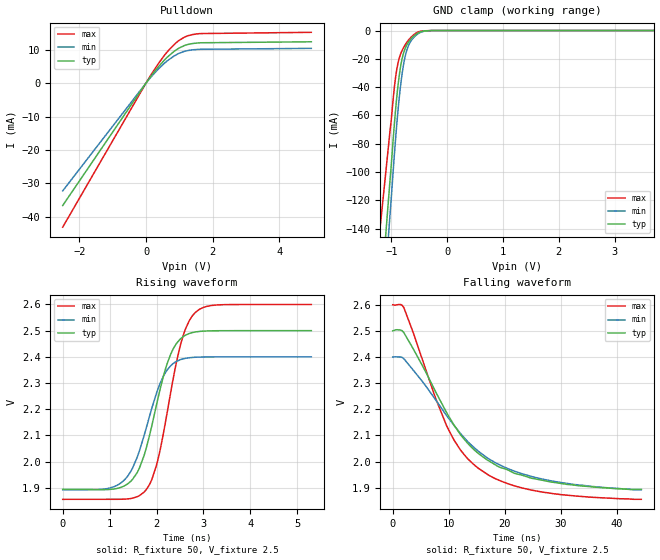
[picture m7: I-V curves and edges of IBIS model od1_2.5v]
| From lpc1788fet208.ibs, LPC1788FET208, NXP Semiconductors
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[Model]   od1_2.5v
Model_type I/O_open_drain
Vinl=7.500E-01
Vinh=1.750E+00
Vref=2.500E+00
Rref=2.000E+03
Cref=0.000E+00
Vmeas=1.250E+00
C_comp   1.240E-12   1.180E-12   1.300E-12
[Voltage Range]   2.500E+00   2.400E+00   2.600E+00
[POWER Clamp Reference]   2.500E+00   2.400E+00   2.600E+00
[GND Clamp Reference]   0.000E+00   0.000E+00   0.000E+00
[Pullup Reference]   2.500E+00   2.400E+00   2.600E+00
[Pulldown Reference]   0.000E+00   0.000E+00   0.000E+00
[Temperature Range]   25   85   -40
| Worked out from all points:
|   slope of the pulldown table from 0 to 0.375 V, typ, clamps not added: 76.6 ohm
|   GND clamp passes 1 mA (typ) near -0.48 V on its own axis
|   rising waveform, R_fixture 50, V_fixture 2.5: 20-80 % time 518ps typ, 542ps min, 493ps max; typ from 1.89 V to 2.5 V
|   falling waveform, R_fixture 50, V_fixture 2.5: 20-80 % time 11.3ns typ, 12.9ns min, 9.37ns max; typ from 2.5 V to 1.89 V
[GND Clamp]
-2.5V     -845.8mA   -925.4mA   -639.1mA
-1.024V   -105mA     -129.3mA   -70.29mA
-944.2mV  -64.53mA   -86.02mA   -38.91mA
-904.3mV  -46.93mA   -66.19mA   -27.41mA
-864.4mV  -33.01mA   -49.12mA   -20.1mA
-804.5mV  -19.17mA   -29.33mA   -13.7mA
-764.6mV  -13.76mA   -20.19mA   -10.79mA
-704.8mV  -8.784mA   -11.65mA   -7.28mA
-645mV    -5.723mA   -7.09mA    -4.61mA
-545.2mV  -2.243mA   -2.909mA   -1.482mA
-246mV    0A         0A         0A
5V        0A         0A         0A
[Pulldown]
-2.5V     -36.61mA   -32.23mA   -43.08mA
172.9mV   2.386mA    2.077mA    2.845mA
611.7mV   7.486mA    6.438mA    9.04mA
930.8mV   10.09mA    8.595mA    12.29mA
1.25V     11.52mA    9.708mA    14.13mA
1.609V    12.03mA    10.08mA    14.78mA
4.96V     12.34mA    10.38mA    15.17mA
[Rising Waveform]
R_fixture = 50
V_fixture = 2.5
V_fixture_min = 2.4
V_fixture_max = 2.6
0s        1.894V     1.893V     1.856V
1.25ns    1.902V     1.92V      1.856V
1.585ns   1.957V     2.015V     1.865V
1.783ns   2.053V     2.13V      1.893V
2.031ns   2.242V     2.277V     2.008V
2.3ns     2.409V     2.366V     2.262V
2.576ns   2.478V     2.393V     2.486V
2.7ns     2.489V     2.397V     2.539V
2.9ns     2.497V     2.399V     2.58V
5.301ns   2.5V       2.4V       2.6V
[Falling Waveform]
R_fixture = 50
V_fixture = 2.5
V_fixture_min = 2.4
V_fixture_max = 2.6
0s        2.5V       2.4V       2.6V
1.948ns   2.494V     2.394V     2.59V
7.691ns   2.266V     2.236V     2.24V
9.589ns   2.189V     2.177V     2.139V
12.04ns   2.105V     2.11V      2.047V
15.03ns   2.036V     2.044V     1.979V
18.93ns   1.98V      1.99V      1.929V
24.72ns   1.937V     1.944V     1.891V
32.45ns   1.91V      1.913V     1.869V
44.4ns    1.894V     1.893V     1.856V
[Ramp]
dV/dt_r   3.6354E-01/5.1510E-10   3.0443E-01/5.3810E-10   4.4652E-01/4.9250E-10
dV/dt_f   3.6354E-01/1.1265E-08   3.0443E-01/1.2924E-08   4.4652E-01/9.3583E-09
R_load = 50
